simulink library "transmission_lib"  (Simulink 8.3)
settings: Solver=ode45  StartTime=0.0  StopTime=10.0  RelTol=1e-3
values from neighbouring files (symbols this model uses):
  dual_clutch = class_REVS_dual_clutch    [class_REVS_DCT_transmission.m]
  electric = class_REVS_electric(engine)    [electric_standard_car.m]
  gear = class_REVS_gearbox    [class_REVS_AMT_transmission.m]    (also in class_REVS_AT_transmission.m; class_REVS_CVT_transmission.m)
  torque_converter = class_REVS_torque_converter    [class_REVS_AT_transmission.m]    (also in class_REVS_CVT_transmission.m)
  transmission = class_REVS_AT_transmission    [transmission_6AT.m]    (also in transmission_8DCT.m = class_REVS_DCT_transmission; transmission_CVT.m = class_REVS_CVT_transmission)
undefined symbols (not defined in the file or in its folder): clutch, convert, gear_strategy, InitialSpeed_radps, LoadSource, SpeedSource, Value
libraries: general_lib x129, simulink x57, transmission_lib x50, audit_lib x11
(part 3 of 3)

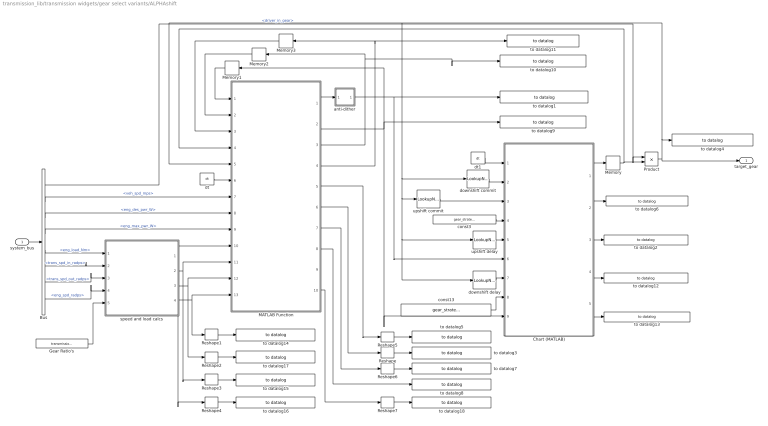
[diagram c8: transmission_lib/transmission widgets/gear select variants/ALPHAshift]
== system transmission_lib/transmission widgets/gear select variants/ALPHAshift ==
  system_bus : Inport
  Bus : BusSelector  OutputSignals=driver.driver_in_gear,vehicle.veh_spd_mps,powertrain.engine.eng_des_pwr_W,powertrain.engine.eng_max_pwr_W,powertrain.engine.eng_load_Nm,powertrain.trans.core.trans_spd_in_radps,powertrain.trans.core.trans_spd_out_radps,powertrain.engine.eng_spd_radps
  Chart (MATLAB) : Stateflow chart  TreatAsAtomicUnit=on
  Gear Ratio's : Constant  Value=transmission.gear.ratio  VectorParams1D=off
  MATLAB Function : MATLAB Function  TreatAsAtomicUnit=on
  Memory{,1..3} (4 alike) : Memory
  Product : Product
  Reshape{,1..7} (8 alike) : Reshape
  anti-dither : Subsystem
  const13 : Constant  Value=gear_strategy.disable_cost_saving_downshifts
  const3 : Constant  Value=gear_strategy.launch_gear_num
  downshift commit : LookupNDDirect  NumberOfTableDimensions=1  Table=gear_strategy.downshift_commit_secs
  downshift delay : LookupNDDirect  NumberOfTableDimensions=1  Table=gear_strategy.downshift_delay_secs
  dt : general_lib/dt
  dt1 : general_lib/dt
  speed and load calcs : Subsystem
  to datalog1 : general_lib/to datalog  VarName=ALPHAshift.desired_gear_num  WorkspaceName=datalog__ALPHAshift__desired_gear_num  VerboseLevel=1  VerboseSignal=REVS.verbose
  to datalog10 : general_lib/to datalog  VarName=ALPHAshift.kickdown_timer  WorkspaceName=datalog__ALPHAshift__kickdown_timer  VerboseLevel=2  VerboseSignal=REVS.verbose
  to datalog11 : general_lib/to datalog  VarName=ALPHAshift.kickdown_ratio  WorkspaceName=datalog__ALPHAshift__kickdown_ratio  VerboseLevel=2  VerboseSignal=REVS.verbose
  to datalog12 : general_lib/to datalog  VarName=ALPHAshift.shift_delay_timer  WorkspaceName=datalog__ALPHAshift__shift_delay_timer  VerboseLevel=2  VerboseSignal=REVS.verbose
  to datalog13 : general_lib/to datalog  VarName=ALPHAshift.in_gear_timer  WorkspaceName=datalog__ALPHAshift__in_gear_timer  VerboseLevel=2  VerboseSignal=REVS.verbose
  to datalog14 : general_lib/to datalog  VarName=ALPHAshift.gear_avail_torque_Nm  WorkspaceName=datalog__ALPHAshift__gear_avail_torque_Nm  VerboseLevel=2  VerboseSignal=REVS.verbose
  to datalog15 : general_lib/to datalog  VarName=ALPHAshift.gear_speed_radps  WorkspaceName=datalog__ALPHAshift__gear_speed_radps  VerboseLevel=2  VerboseSignal=REVS.verbose
  to datalog16 : general_lib/to datalog  VarName=ALPHAshift.gear_torque_Nm  WorkspaceName=datalog__ALPHAshift__gear_torque_Nm  VerboseLevel=2  VerboseSignal=REVS.verbose
  to datalog17 : general_lib/to datalog  VarName=ALPHAshift.gear_cost  WorkspaceName=datalog__ALPHAshift__gear_cost  VerboseLevel=2  VerboseSignal=REVS.verbose
  to datalog18 : general_lib/to datalog  VarName=ALPHAshift.kickdown_disability_code  WorkspaceName=datalog__ALPHAshift__kickdown_disability_code  VerboseLevel=2  VerboseSignal=REVS.verbose
  to datalog2 : general_lib/to datalog  VarName=ALPHAshift.shift_reason  WorkspaceName=datalog__ALPHAshift__shift_reason  VerboseLevel=1  VerboseSignal=REVS.verbose
  to datalog3 : general_lib/to datalog  VarName=ALPHAshift.disability_code  WorkspaceName=datalog__ALPHAshift__disability_code  VerboseLevel=2  VerboseSignal=REVS.verbose
  to datalog4 : general_lib/to datalog  VarName=ALPHAshift.current_gear_num  WorkspaceName=datalog__ALPHAshift__current_gear_num  VerboseLevel=1  VerboseSignal=REVS.verbose
  to datalog5 : general_lib/to datalog  VarName=ALPHAshift.gear_available  WorkspaceName=datalog__ALPHAshift__gear_available  VerboseLevel=2  VerboseSignal=REVS.verbose
  to datalog6 : general_lib/to datalog  VarName=ALPHAshift.shift_type  WorkspaceName=datalog__ALPHAshift__shift_type  VerboseLevel=1  VerboseSignal=REVS.verbose
  to datalog7 : general_lib/to datalog  VarName=ALPHAshift.better_fuel_gear  WorkspaceName=datalog__ALPHAshift__better_fuel_gear  VerboseLevel=1  VerboseSignal=REVS.verbose
  to datalog8 : general_lib/to datalog  VarName=ALPHAshift.min_fuel_gear  WorkspaceName=datalog__ALPHAshift__min_fuel_gear  VerboseLevel=1  VerboseSignal=REVS.verbose
  to datalog9 : general_lib/to datalog  VarName=ALPHAshift.desired_shift_reason  WorkspaceName=datalog__ALPHAshift__desired_shift_reason  VerboseLevel=1  VerboseSignal=REVS.verbose
  upshift commit : LookupNDDirect  NumberOfTableDimensions=1  Table=gear_strategy.upshift_commit_secs
  upshift delay : LookupNDDirect  NumberOfTableDimensions=1  Table=gear_strategy.upshift_delay_secs
  target_gear : Outport
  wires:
  Reshape6/1 -> to datalog7/1
  Reshape5/1 -> to datalog5/1
  MATLAB Function/1(desired_gear_num) -> anti-dither/1(raw)
  anti-dither/1(out) -> Chart (MATLAB)/6(desired_gear_num), to datalog1/1
  Reshape1/1 -> to datalog14/1
  Reshape3/1 -> to datalog15/1
  Reshape4/1 -> to datalog16/1
  Reshape/1 -> to datalog3/1
  speed and load calcs/4(gear_avail_trq_Nm) -> MATLAB Function/13(gear_avail_trq_Nm), Reshape1/1
  MATLAB Function/8(min_cost_gear) -> to datalog8/1
  MATLAB Function/7(better_cost_gear) -> Reshape6/1
  Chart (MATLAB)/1(command_gear_num) -> Memory/1
  Bus/2 -> MATLAB Function/7(vehicle_spd_mps)  "<veh_spd_mps>"
  dt/1 -> MATLAB Function/6(dt)
  speed and load calcs/3(gear_cost) -> Reshape2/1, MATLAB Function/12(gear_cost)
  system_bus/1 -> Bus/1
  Product/1 -> target_gear/1, to datalog4/1, downshift delay/1, upshift delay/1, upshift commit/1, downshift commit/1, MATLAB Function/5(current_gear_num)
  Chart (MATLAB)/3(shift_reason) -> to datalog2/1
  MATLAB Function/6(gear_disability_code) -> Reshape/1
  MATLAB Function/5(gear_available) -> Reshape5/1
  Chart (MATLAB)/2(previous_shift_type) -> to datalog6/1
  Bus/3 -> MATLAB Function/8(driver_des_pwr_W)  "<eng_des_pwr_W>"
  Bus/4 -> MATLAB Function/9(engine_max_pwr_W)  "<eng_max_pwr_W>"
  Memory/1 -> Product/2, MATLAB Function/4(command_gear_num)
  Bus/1 -> Product/1  "<driver_in_gear>"
  dt1/1 -> Chart (MATLAB)/1(dt)
  downshift delay/1 -> Chart (MATLAB)/7(downshift_delay_secs)
  upshift commit/1 -> Chart (MATLAB)/3(upshift_min_duration_secs)
  downshift commit/1 -> Chart (MATLAB)/2(downshift_min_duration_secs)
  upshift delay/1 -> Chart (MATLAB)/5(upshift_delay_secs)
  const13/1 -> Chart (MATLAB)/8(legacy_downshift_mode)
  const3/1 -> Chart (MATLAB)/4(launch_gear_num)
  MATLAB Function/2(desired_shift_reason) -> Chart (MATLAB)/9(desired_shift_reason), Memory1/1, to datalog9/1
  Memory1/1 -> MATLAB Function/1(desired_shift_reason_prev)
  MATLAB Function/3(kickdown_timer) -> to datalog10/1, Memory2/1
  Memory2/1 -> MATLAB Function/2(kickdown_timer_prev)
  Memory3/1 -> MATLAB Function/3(kickdown_ratio_prev)
  MATLAB Function/4(kickdown_ratio) -> Memory3/1, to datalog11/1
  speed and load calcs/2(gear_spd_radps) -> MATLAB Function/11(gear_spd_radps), Reshape3/1
  Bus/5 -> speed and load calcs/1(eng_load_Nm)  "<eng_load_Nm>"
  Bus/6 -> speed and load calcs/2(trans_spd_in_radps)  "<trans_spd_in_radps>"
  Bus/7 -> speed and load calcs/3(trans_spd_out_radps)  "<trans_spd_out_radps>"
  Bus/8 -> speed and load calcs/4(eng_spd_radps)  "<eng_spd_radps>"
  Gear Ratio's/1 -> speed and load calcs/5(trans_gear_ratios)
  speed and load calcs/1(gear_trq_Nm) -> MATLAB Function/10(gear_trq_Nm), Reshape4/1
  Chart (MATLAB)/4(shift_delay_timer) -> to datalog12/1
  Chart (MATLAB)/5(in_gear_timer) -> to datalog13/1
  Reshape2/1 -> to datalog17/1
  Reshape7/1 -> to datalog18/1
  MATLAB Function/10(kickdown_disability_code) -> Reshape7/1

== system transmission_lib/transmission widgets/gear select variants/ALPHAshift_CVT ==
  system_bus : Inport
  Bus Selector : BusSelector  OutputSignals=powertrain.trans.core.trans_spd_out_radps,driver.driver_in_gear,powertrain.engine.eng_des_pwr_W
  MinMax : MinMax  Function=max  Inputs=2
  Product2 : Product  Inputs=**
  Product4 : Product  Inputs=*/
  Saturation5 : Saturate  UpperLimit=max(transmission.gear.ratio)  LowerLimit=min(transmission.gear.ratio(2:end))
  Transfer Fcn : TransferFcn  Denominator=[0.0 1]
  eps : Saturate  UpperLimit=Inf  LowerLimit=eps
  min BSFC speed : Lookup_n-D  NumberOfTableDimensions=1  BreakpointsForDimension1=transmission.gear_strategy.min_bsfc_power_W  Table=transmission.gear_strategy.min_bsfc_speed_rapds  ExtrapMethod=Clip  InternalRulePriority=Speed  RndMeth=Simplest
  min speed table : general_lib/dynamic lookup  LookupStructure=transmission.gear_strategy.min_speed_radps  InterpMethod=Linear  ExtrapMethod=Clip  DiagnosticForOutOfRangeInput=Warning  IndexSearchMethod=Linear search  BeginIndexSearchUsingPreviousIndexResult=on  SupportTunableTableSize=off  LookupStructureEval=|
      | LookupStructure =
      | 
      |      []
  to datalog1 : general_lib/to datalog  VarName=cvtshift.target_ratio  WorkspaceName=datalog__cvtshift__target_ratio  VerboseLevel=3  VerboseSignal=REVS.verbose
  to datalog8 : general_lib/to datalog  VarName=cvtshift.target_speed_radps  WorkspaceName=datalog__cvtshift__target_speed_radps  VerboseLevel=3  VerboseSignal=REVS.verbose
  target_gear : Outport
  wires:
  system_bus/1 -> min speed table/1, Bus Selector/1
  Bus Selector/1 -> eps/1  "<trans_spd_out_radps>"
  Bus Selector/3 -> min BSFC speed/1  "<eng_des_pwr_W>"
  Product4/1 -> Saturation5/1
  Saturation5/1 -> Product2/2
  eps/1 -> Product4/2
  Bus Selector/2 -> Product2/1  "<driver_in_gear>"
  Product2/1 -> Transfer Fcn/1
  Transfer Fcn/1 -> to datalog1/1, target_gear/1
  min BSFC speed/1 -> MinMax/1
  min speed table/1 -> MinMax/2
  MinMax/1 -> to datalog8/1, Product4/1

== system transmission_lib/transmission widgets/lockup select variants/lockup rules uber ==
  gear_number : Inport
  system_bus : Inport  Port=2
  Bus Creator1 : BusCreator  Inputs=3
  Data Type Conversion : DataTypeConversion
  Detect Decrease : simulink/Logic and Bit Operations/Detect Decrease  vinit=0.0  InputProcessing=Inherited  OutDataTypeStr=boolean
  Detect Increase : simulink/Logic and Bit Operations/Detect Increase  vinit=0.0  InputProcessing=Inherited  OutDataTypeStr=boolean
  Logical Operator2 : Logic  Operator=NAND  AllPortsSameDT=off  OutDataTypeStr=boolean
  Logical Operator3 : Logic  Operator=NOT  AllPortsSameDT=off  OutDataTypeStr=boolean
  Logical Operator6 : Logic  Operator=NAND  AllPortsSameDT=off  OutDataTypeStr=boolean
  Logical Operator8 : Logic  Operator=OR  AllPortsSameDT=off  OutDataTypeStr=boolean
  Logical Operator9 : Logic  Inputs=5  AllPortsSameDT=off  OutDataTypeStr=boolean
  Memory : Memory
  Relational Operator : RelationalOperator  Operator=>  OutDataTypeStr=boolean  ZeroCross=off
  boolean integrator : general_lib/boolean integrator  UpperSaturationLimit=Inf  Normalize=off
  const1 : Constant  Value=transmission.tcc_strategy.lockup_allowed
  const3 : Constant  Value=transmission.tcc_strategy.lockup_delay_secs
  downshift unlock criteria : general_lib/dynamic equation  DynamicExpression=transmission.tcc_strategy.downshift_unlock_condition  DynamicExpressionEval=0
  lockup criteria : general_lib/dynamic equation  DynamicExpression=transmission.tcc_strategy.lock_condition  DynamicExpressionEval=(@gb_spd_out_radps > @table_lock_spd && @trans_curr_gear > transmission.tcc_strategy.always_unlock_gear ) || @trans_curr_gear >= transmission.tcc_strategy.always_lock_gear
  lockup table : general_lib/dynamic lookup  LookupStructure=transmission.tcc_strategy.lock_table  InterpMethod=Linear  ExtrapMethod=Clip  DiagnosticForOutOfRangeInput=Warning  IndexSearchMethod=Linear search  BeginIndexSearchUsingPreviousIndexResult=on  SupportTunableTableSize=off  LookupStructureEval=|
      | LookupStructure =
      | 
      |      []
  unlock criteria : general_lib/dynamic equation  DynamicExpression=transmission.tcc_strategy.unlock_condition  DynamicExpressionEval=(@gb_spd_out_radps < @table_unlock_spd && @trans_curr_gear < transmission.tcc_strategy.always_lock_gear ) || @trans_curr_gear <= transmission.tcc_strategy.always_unlock_gear
  unlock table : general_lib/dynamic lookup  LookupStructure=transmission.tcc_strategy.unlock_table  InterpMethod=Linear  ExtrapMethod=Clip  DiagnosticForOutOfRangeInput=Warning  IndexSearchMethod=Linear search  BeginIndexSearchUsingPreviousIndexResult=on  SupportTunableTableSize=off  LookupStructureEval=|
      | LookupStructure =
      | 
      |      []
  upshift unlock criteria : general_lib/dynamic equation  DynamicExpression=transmission.tcc_strategy.upshift_unlock_condition  DynamicExpressionEval=0
  lockup_cmd : Outport
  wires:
  Logical Operator6/1 -> Logical Operator9/2
  Logical Operator2/1 -> Logical Operator9/3
  Detect Increase/1 -> Logical Operator2/2
  system_bus/1 -> Bus Creator1/3, unlock table/1, lockup table/1, upshift unlock criteria/1, downshift unlock criteria/1  "system_bus"
  Logical Operator9/1 -> boolean integrator/1
  Logical Operator8/1 -> Logical Operator9/4
  const3/1 -> Relational Operator/2
  Detect Decrease/1 -> Logical Operator6/2
  gear_number/1 -> Detect Increase/1, Detect Decrease/1
  boolean integrator/1 -> Relational Operator/1
  const1/1 -> Logical Operator9/1
  Relational Operator/1 -> Data Type Conversion/1
  Data Type Conversion/1 -> lockup_cmd/1, Memory/1  "tcc_lockup_cmd_bool"
  unlock criteria/1 -> Logical Operator3/1
  downshift unlock criteria/1 -> Logical Operator6/1
  upshift unlock criteria/1 -> Logical Operator2/1
  Logical Operator3/1 -> Logical Operator9/5
  lockup table/1 -> Bus Creator1/1  "table_lock_spd"
  Bus Creator1/1 -> lockup criteria/1, unlock criteria/1
  unlock table/1 -> Bus Creator1/2  "table_unlock_spd"
  lockup criteria/1 -> Logical Operator8/2
  Memory/1 -> Logical Operator8/1

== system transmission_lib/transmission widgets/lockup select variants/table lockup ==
  gear_number : Inport
  system_bus : Inport  Port=2
  const : Constant  Value=transmission.tcc_strategy.lockup_allowed
  const2 : Constant  Value=transmission.tcc_strategy.lockup_delay_secs
  dt : general_lib/dt
  "lock map " : Lookup_n-D  BreakpointsForDimension1=transmission.tcc_strategy.lock_map_load  BreakpointsForDimension2=transmission.gear.number(2:end)  Table=transmission.tcc_strategy.lock_map_speed  RndMeth=Simplest
  lockup load select : transmission_lib/transmission widgets/load select  LoadSource=transmission.tcc_strategy.lockup_load_source
  lockup speed select : transmission_lib/transmission widgets/speed select  SpeedSource=transmission.tcc_strategy.lockup_speed_source
  tcc lockup : Stateflow chart  TreatAsAtomicUnit=on
  "unlock map " : Lookup_n-D  BreakpointsForDimension1=transmission.tcc_strategy.unlock_map_load  BreakpointsForDimension2=transmission.gear.number(2:end)  Table=transmission.tcc_strategy.unlock_map_speed  RndMeth=Simplest
  lockup_cmd : Outport
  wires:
  dt/1 -> tcc lockup/2(step_time)
  lockup speed select/1 -> tcc lockup/1(lock_spd)
  "unlock map "/1 -> tcc lockup/4(release_spd)
  "lock map "/1 -> tcc lockup/3(lockup_spd)
  tcc lockup/1(tcc_lockup) -> lockup_cmd/1  "tcc_lockup_cmd_bool"
  const/1 -> tcc lockup/5(lockup_allowed)
  lockup load select/1 -> "unlock map "/1, "lock map "/1
  const2/1 -> tcc lockup/6(lockup_delay_secs)
  system_bus/1 -> lockup load select/1, lockup speed select/1
  gear_number/1 -> "lock map "/2, "unlock map "/2

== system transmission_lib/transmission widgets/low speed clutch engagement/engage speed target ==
  curr : Inport
  Constant : Constant  Value=clutch.engage_speed_radps(1)
  Constant1 : Constant  Value=clutch.engage_speed_radps(end)
  Divide : Product  Inputs=*/
  Interp 0-1 : general_lib/Interp 0-1
  tgt : Outport
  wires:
  Constant/1 -> Interp 0-1/2
  Constant1/1 -> Interp 0-1/3, Divide/2
  Divide/1 -> Interp 0-1/1
  curr/1 -> Divide/1
  Interp 0-1/1 -> tgt/1

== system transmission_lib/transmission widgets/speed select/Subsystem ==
  veh_spd_mps : Inport
  Axle Speed (rad/sec) : Product  Inputs=/*
  Non Zero : Saturate  UpperLimit=Inf  LowerLimit=eps  ZeroCross=off
  Tire Radius (m) : Constant  Value=vehicle.drive_axle1.tire.radius_m
  wheel_spd_radps : Outport
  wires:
  Tire Radius (m)/1 -> Non Zero/1
  Axle Speed (rad/sec)/1 -> wheel_spd_radps/1
  Non Zero/1 -> Axle Speed (rad/sec)/1
  veh_spd_mps/1 -> Axle Speed (rad/sec)/2

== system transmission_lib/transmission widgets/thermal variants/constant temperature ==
  system_bus : Inport
  Bus Creator : BusCreator  Inputs=1
  Constant : Constant  Value=transmission.thermal.temperature_degC
  thermal_bus : Outport
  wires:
  Constant/1 -> Bus Creator/1  "trans_temp_degC"
  Bus Creator/1 -> thermal_bus/1

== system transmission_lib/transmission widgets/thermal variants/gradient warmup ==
  system_bus : Inport
  Bus Creator : BusCreator  Inputs=1
  Constant : Constant  Value=transmission.thermal.final_temperature_degC
  State-Space : StateSpace  A=-1/transmission.thermal.gradient_time_constant_sec  C=1/transmission.thermal.gradient_time_constant_sec  D=0  X0=transmission.thermal.initial_temperature_degC  ContinuousStateAttributes='temperature'
  thermal_bus : Outport
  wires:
  State-Space/1 -> Bus Creator/1  "trans_temp_degC"
  Bus Creator/1 -> thermal_bus/1
  Constant/1 -> State-Space/1

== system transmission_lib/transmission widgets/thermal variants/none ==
  system_bus : Inport
  thermal_bus : Outport

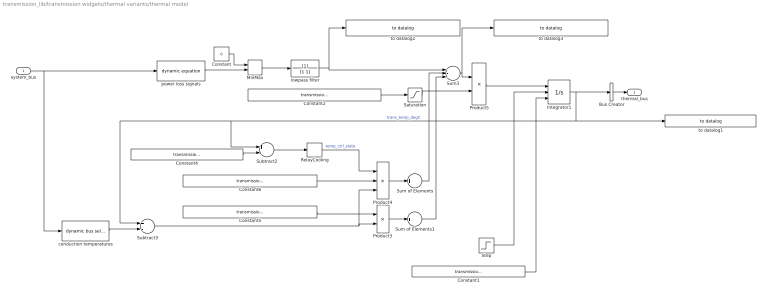
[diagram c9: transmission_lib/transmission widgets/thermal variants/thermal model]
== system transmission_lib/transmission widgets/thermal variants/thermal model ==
  system_bus : Inport
  Bus Creator : BusCreator  Inputs=1
  Constant : Constant  Value=0
  Constant1 : Constant  Value=transmission.thermal.initial_temperature_degC
  Constant2 : Constant  Value=transmission.thermal.capacity_JpK
  Constant4 : Constant  Value=transmission.thermal.target_temperature_degC
  Constant5 : Constant  Value=transmission.thermal.passive_conductance_WpK
  Constant6 : Constant  Value=transmission.thermal.cooling_conductance_WpK
  Integrator1 : Integrator  ExternalReset=level  InitialConditionSource=external  InitialCondition=transmission.thermal.initial_temperature_degC  ZeroCross=off
  MinMax : MinMax  Function=max  Inputs=2
  Product3 : Product  Inputs=**
  Product4 : Product  Inputs=***
  Product5 : Product  Inputs=*/
  RelayCooling : Relay  OnSwitchValue=1  OffSwitchValue=-1  ZeroCross=off
  Saturation : Saturate  UpperLimit=Inf  LowerLimit=eps
  Step : Step  Before=1  After=0  SampleTime=0  ZeroCross=off
  Subtract2 : Sum  Inputs=+-
  Subtract3 : Sum  Inputs=+-
  Sum of Elements : Sum  Inputs=+
  Sum of Elements1 : Sum  Inputs=+
  Sum3 : Sum  Inputs=+--
  conduction temperatures : general_lib/dynamic bus select  SignalList=transmission.thermal.conduction_temperatures
  lowpass filter : TransferFcn  Denominator=[1 1]
  power loss signals : general_lib/dynamic equation  DynamicExpression=transmission.thermal.power_loss_expr
  to datalog1 : general_lib/to datalog  VarName=transmission.temperature_C  WorkspaceName=datalog__transmission__temperature_C  VerboseLevel=2  VerboseSignal=REVS.verbose
  to datalog2 : general_lib/to datalog  VarName=transmission.thermal_loss_power_input_W  WorkspaceName=datalog__transmission__thermal_loss_power_input_W  VerboseLevel=2  VerboseSignal=REVS.verbose
  to datalog3 : general_lib/to datalog  VarName=transmission.thermal_net_power_W  WorkspaceName=datalog__transmission__thermal_net_power_W  VerboseLevel=2  VerboseSignal=REVS.verbose
  thermal_bus : Outport
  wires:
  Product4/1 -> Sum of Elements/1
  Product3/1 -> Sum of Elements1/1
  Sum of Elements/1 -> Sum3/2
  Sum of Elements1/1 -> Sum3/3
  Constant6/1 -> Product4/2
  Constant5/1 -> Product3/1
  Subtract3/1 -> Product3/2, Product4/3
  conduction temperatures/1 -> Subtract3/2
  Constant/1 -> MinMax/1
  power loss signals/1 -> MinMax/2
  system_bus/1 -> conduction temperatures/1, power loss signals/1
  lowpass filter/1 -> Sum3/1, to datalog2/1
  Product5/1 -> Integrator1/1
  Sum3/1 -> Product5/1, to datalog3/1
  Integrator1/1 -> Bus Creator/1, Subtract2/1, Subtract3/1, to datalog1/1  "trans_temp_degC"
  Constant2/1 -> Saturation/1
  Saturation/1 -> Product5/2
  MinMax/1 -> lowpass filter/1
  Bus Creator/1 -> thermal_bus/1
  Constant4/1 -> Subtract2/2
  RelayCooling/1 -> Product4/1  "temp_ctrl_state"
  Subtract2/1 -> RelayCooling/1
  Constant1/1 -> Integrator1/3
  Step/1 -> Integrator1/2

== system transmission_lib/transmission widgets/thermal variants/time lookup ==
  system_bus : Inport
  1-D Lookup Table : Lookup_n-D  NumberOfTableDimensions=1  BreakpointsForDimension1=transmission.thermal.temperature_time_sec  IndexSearchMethod=Linear search  BeginIndexSearchUsingPreviousIndexResult=on  Table=transmission.thermal.temperature_degC  ExtrapMethod=Clip  InternalRulePriority=Speed  RndMeth=Simplest
  Bus Creator : BusCreator  Inputs=1
  Bus Selector : BusSelector  OutputSignals=driver.cycle_pos_secs
  thermal_bus : Outport
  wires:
  Bus Selector/1 -> 1-D Lookup Table/1  "<cycle_pos_secs>"
  1-D Lookup Table/1 -> Bus Creator/1  "trans_temp_degC"
  Bus Creator/1 -> thermal_bus/1
  system_bus/1 -> Bus Selector/1

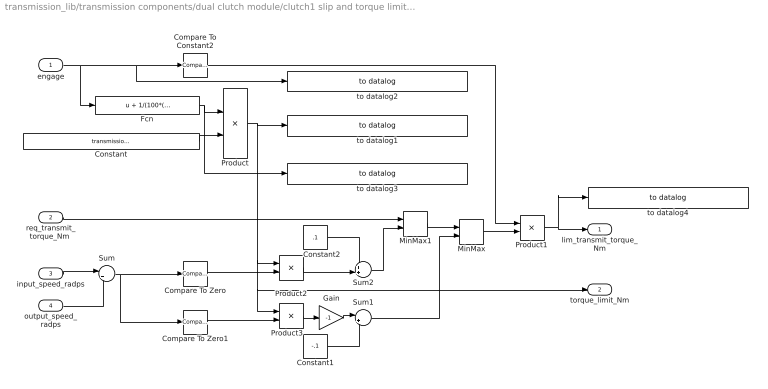
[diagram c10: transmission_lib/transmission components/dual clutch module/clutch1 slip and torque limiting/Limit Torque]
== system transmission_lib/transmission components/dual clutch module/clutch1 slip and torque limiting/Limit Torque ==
  engage : Inport
  "req_transmit_torque_Nm " : Inport  Port=2
  input_speed_radps : Inport  Port=3
  output_speed_radps : Inport  Port=4
  Compare To Constant2 : simulink/Logic and Bit Operations/Compare To Constant  relop=>  const=0  OutDataTypeStr=boolean
  Compare To Zero : simulink/Logic and Bit Operations/Compare To Zero  relop=>=  OutDataTypeStr=boolean  ZeroCross=off
  Compare To Zero1 : simulink/Logic and Bit Operations/Compare To Zero  relop=<=  OutDataTypeStr=boolean  ZeroCross=off
  Constant : Constant  Value=transmission.dual_clutch.torque_capacity_Nm
  Constant1 : Constant  Value=-.1
  Constant2 : Constant  Value=.1
  Fcn : Fcn  Expr=u + 1/(100*(1+eps-u))
  Gain : Gain  Gain=-1
  MinMax : MinMax  Function=max  Inputs=2  ZeroCross=off
  MinMax1 : MinMax  Inputs=2  ZeroCross=off
  Product{,1..3} (4 alike) : Product
  Sum : Sum  Inputs=|+-
  Sum1 : Sum  Inputs=|++
  Sum2 : Sum  Inputs=++|
  to datalog1 : general_lib/to datalog  VarName=transmission__clutch1_torque_limit_Nm  WorkspaceName=datalog__transmission__clutch1_torque_limit_Nm  VerboseLevel=3  VerboseSignal=REVS.verbose
  to datalog2 : general_lib/to datalog  VarName=transmission__clutch1_engage  WorkspaceName=datalog__transmission__clutch1_engage  VerboseLevel=1  VerboseSignal=REVS.verbose
  to datalog3 : general_lib/to datalog  VarName=transmission__clutch1_capacity_norm  WorkspaceName=datalog__transmission__clutch1_capacity_norm  VerboseLevel=3  VerboseSignal=REVS.verbose
  to datalog4 : general_lib/to datalog  VarName=transmission__clutch1_torque_Nm  WorkspaceName=datalog__transmission__clutch1_torque_Nm  VerboseLevel=3  VerboseSignal=REVS.verbose
  lim_transmit_torque_Nm : Outport
  torque_limit_Nm : Outport  Port=2
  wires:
  Fcn/1 -> Product/1, to datalog3/1
  Sum2/1 -> MinMax1/2
  Product3/1 -> Gain/1
  Constant2/1 -> Sum2/1
  Product2/1 -> Sum2/2
  Compare To Zero1/1 -> Product3/2
  Compare To Zero/1 -> Product2/2
  Sum/1 -> Compare To Zero/1, Compare To Zero1/1
  Sum1/1 -> MinMax/2
  Constant1/1 -> Sum1/2
  output_speed_radps/1 -> Sum/2
  input_speed_radps/1 -> Sum/1
  "req_transmit_torque_Nm "/1 -> MinMax1/1
  Gain/1 -> Sum1/1
  MinMax1/1 -> MinMax/1
  Constant/1 -> Product/2
  engage/1 -> Fcn/1, Compare To Constant2/1, to datalog2/1
  Product/1 -> to datalog1/1, torque_limit_Nm/1, Product3/1, Product2/1
  MinMax/1 -> Product1/2
  Product1/1 -> lim_transmit_torque_Nm/1, to datalog4/1
  Compare To Constant2/1 -> Product1/1

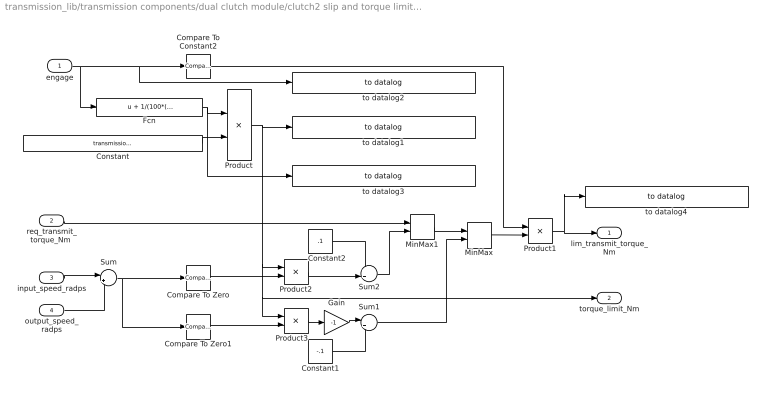
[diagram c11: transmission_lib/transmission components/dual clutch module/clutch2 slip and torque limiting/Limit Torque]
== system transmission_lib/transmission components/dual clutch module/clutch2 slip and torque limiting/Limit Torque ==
  engage : Inport
  "req_transmit_torque_Nm " : Inport  Port=2
  input_speed_radps : Inport  Port=3
  output_speed_radps : Inport  Port=4
  Compare To Constant2 : simulink/Logic and Bit Operations/Compare To Constant  relop=>  const=0  OutDataTypeStr=boolean
  Compare To Zero : simulink/Logic and Bit Operations/Compare To Zero  relop=>=  OutDataTypeStr=boolean  ZeroCross=off
  Compare To Zero1 : simulink/Logic and Bit Operations/Compare To Zero  relop=<=  OutDataTypeStr=boolean  ZeroCross=off
  Constant : Constant  Value=transmission.dual_clutch.torque_capacity_Nm
  Constant1 : Constant  Value=-.1
  Constant2 : Constant  Value=.1
  Fcn : Fcn  Expr=u + 1/(100*(1+eps-u))
  Gain : Gain  Gain=-1
  MinMax : MinMax  Function=max  Inputs=2  ZeroCross=off
  MinMax1 : MinMax  Inputs=2  ZeroCross=off
  Product{,1..3} (4 alike) : Product
  Sum : Sum  Inputs=|+-
  Sum1 : Sum  Inputs=|++
  Sum2 : Sum  Inputs=++|
  to datalog1 : general_lib/to datalog  VarName=transmission__clutch2_torque_limit_Nm  WorkspaceName=datalog__transmission__clutch2_torque_limit_Nm  VerboseLevel=3  VerboseSignal=REVS.verbose
  to datalog2 : general_lib/to datalog  VarName=transmission__clutch2_engage  WorkspaceName=datalog__transmission__clutch2_engage  VerboseLevel=1  VerboseSignal=REVS.verbose
  to datalog3 : general_lib/to datalog  VarName=transmission__clutch2_capacity_norm  WorkspaceName=datalog__transmission__clutch2_capacity_norm  VerboseLevel=3  VerboseSignal=REVS.verbose
  to datalog4 : general_lib/to datalog  VarName=transmission__clutch2_torque_Nm  WorkspaceName=datalog__transmission__clutch2_torque_Nm  VerboseLevel=3  VerboseSignal=REVS.verbose
  lim_transmit_torque_Nm : Outport
  torque_limit_Nm : Outport  Port=2
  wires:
  Fcn/1 -> Product/1, to datalog3/1
  Sum2/1 -> MinMax1/2
  Product3/1 -> Gain/1
  Constant2/1 -> Sum2/1
  Product2/1 -> Sum2/2
  Compare To Zero1/1 -> Product3/2
  Compare To Zero/1 -> Product2/2
  Sum/1 -> Compare To Zero/1, Compare To Zero1/1
  Sum1/1 -> MinMax/2
  Constant1/1 -> Sum1/2
  output_speed_radps/1 -> Sum/2
  input_speed_radps/1 -> Sum/1
  "req_transmit_torque_Nm "/1 -> MinMax1/1
  Gain/1 -> Sum1/1
  MinMax1/1 -> MinMax/1
  Constant/1 -> Product/2
  engage/1 -> Compare To Constant2/1, to datalog2/1, Fcn/1
  Product/1 -> to datalog1/1, torque_limit_Nm/1, Product3/1, Product2/1
  MinMax/1 -> Product1/2
  Product1/1 -> lim_transmit_torque_Nm/1, to datalog4/1
  Compare To Constant2/1 -> Product1/1

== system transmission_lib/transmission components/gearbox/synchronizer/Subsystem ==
  engage : Inport
  spd_out : Inport  Port=2
  spd_in : Inport  Port=3
  Compare To Constant1 : simulink/Logic and Bit Operations/Compare To Constant  relop=<=  const=1e-3  OutDataTypeStr=boolean  ZeroCross=off
  Compare To Constant2 : simulink/Logic and Bit Operations/Compare To Constant  relop=<=  const=1e-3  OutDataTypeStr=boolean  ZeroCross=off
  Compare To Constant3 : simulink/Logic and Bit Operations/Compare To Constant  relop=>  const=0  OutDataTypeStr=boolean  ZeroCross=off
  Compare To Constant4 : simulink/Logic and Bit Operations/Compare To Constant  relop===  const=1  OutDataTypeStr=boolean
  Logical Operator : Logic  Operator=OR  AllPortsSameDT=off  OutDataTypeStr=boolean
  Logical Operator1 : Logic  Inputs=3  AllPortsSameDT=off  OutDataTypeStr=boolean
  Memory2 : Memory
  lockup : Outport
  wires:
  Compare To Constant4/1 -> Logical Operator/1
  Memory2/1 -> Logical Operator/2
  Compare To Constant1/1 -> Logical Operator1/2
  Compare To Constant2/1 -> Logical Operator1/3
  engage/1 -> Compare To Constant3/1, Compare To Constant4/1
  Logical Operator/1 -> lockup/1
  spd_out/1 -> Compare To Constant1/1
  spd_in/1 -> Compare To Constant2/1
  Logical Operator1/1 -> Memory2/1
  Compare To Constant3/1 -> Logical Operator1/1

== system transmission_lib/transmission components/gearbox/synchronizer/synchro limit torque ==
  engage : Inport
  "req_transmit_torque_Nm " : Inport  Port=2
  input_speed_radps : Inport  Port=3
  output_speed_radps : Inport  Port=4
  Compare To Constant2 : simulink/Logic and Bit Operations/Compare To Constant  relop=>  const=0  OutDataTypeStr=boolean
  Compare To Zero : simulink/Logic and Bit Operations/Compare To Zero  relop=>=  OutDataTypeStr=boolean
  Compare To Zero1 : simulink/Logic and Bit Operations/Compare To Zero  relop=<=  OutDataTypeStr=boolean
  Constant : Constant  Value=.1
  Constant1 : Constant  Value=-.1
  Constant2 : Constant  Value=inf
  Constant3 : Constant  Value=-inf
  MinMax : MinMax  Function=max  Inputs=2  ZeroCross=off
  MinMax1 : MinMax  Inputs=2  ZeroCross=off
  Product : Product
  Product1 : Product
  Product2 : Product
  Sum : Sum  Inputs=|+-
  Sum1 : Sum  Inputs=|++
  Sum2 : Sum  Inputs=++|
  lim_transmit_torque_Nm : Outport
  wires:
  Sum2/1 -> MinMax1/2
  Sum/1 -> Compare To Zero/1, Compare To Zero1/1
  Compare To Constant2/1 -> Product1/1
  output_speed_radps/1 -> Sum/2
  input_speed_radps/1 -> Sum/1
  MinMax1/1 -> MinMax/1
  engage/1 -> Compare To Constant2/1
  MinMax/1 -> Product1/2
  "req_transmit_torque_Nm "/1 -> MinMax1/1
  Product1/1 -> lim_transmit_torque_Nm/1
  Sum1/1 -> MinMax/2
  Constant1/1 -> Sum1/2
  Constant/1 -> Sum2/1
  Compare To Zero/1 -> Product/2
  Compare To Zero1/1 -> Product2/1
  Constant3/1 -> Product2/2
  Constant2/1 -> Product/1
  Product2/1 -> Sum1/1
  Product/1 -> Sum2/2

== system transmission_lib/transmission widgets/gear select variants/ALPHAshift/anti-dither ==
  raw : Inport
  Abs : Abs
  Memory : Memory
  Rounding Function : Rounding  Operator=round
  Sum : Sum  Inputs=|+-
  Switch : Switch  Criteria=u2 > Threshold  Threshold=.66
  low pass filter : TransferFcn  Denominator=[0.02 1]
  to datalog17 : general_lib/to datalog  VarName=ALPHAshift.filtered_desired_gear_num  WorkspaceName=datalog__ALPHAshift__filtered_desired_gear_num  VerboseLevel=3  VerboseSignal=REVS.verbose
  to datalog18 : general_lib/to datalog  VarName=ALPHAshift.raw_desired_gear_num  WorkspaceName=datalog__ALPHAshift__raw_desired_gear_num  VerboseLevel=3  VerboseSignal=REVS.verbose
  out : Outport
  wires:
  Abs/1 -> Switch/2
  Memory/1 -> Switch/3, Sum/2
  Sum/1 -> Abs/1
  Switch/1 -> Memory/1, out/1
  Rounding Function/1 -> Switch/1
  low pass filter/1 -> to datalog17/1, Sum/1, Rounding Function/1
  raw/1 -> low pass filter/1, to datalog18/1

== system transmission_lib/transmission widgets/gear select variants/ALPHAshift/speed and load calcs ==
  eng_load_Nm : Inport
  trans_spd_in_radps : Inport  Port=2
  trans_spd_out_radps : Inport  Port=3
  eng_spd_radps : Inport  Port=4
  trans_gear_ratios : Inport  Port=5
  Logical Operator : Logic  Operator=NOT  AllPortsSameDT=off  OutDataTypeStr=boolean
  MinMax : MinMax  Inputs=2  ZeroCross=off
  MinMax1 : MinMax  Function=max  ZeroCross=off
  MinMax2 : MinMax  Function=max  Inputs=2  ZeroCross=off
  Product1 : Product  Inputs=***/
  Product2 : Product  Inputs=***
  Product3 : Product  Inputs=*/
  Product4 : Product  Inputs=***/
  Product5 : Product  Inputs=**
  Sum : Sum  Inputs=|++
  cost map : Lookup_n-D  BreakpointsForDimension1=gear_strategy.cost_map_torque_Nm  BreakpointsForDimension2=gear_strategy.cost_map_speed_radps  IndexSearchMethod=Linear search  BeginIndexSearchUsingPreviousIndexResult=on  Table=gear_strategy.cost_map  ExtrapMethod=Clip  UseLastTableValue=on  RndMeth=Simplest
  eps1 : Saturate  UpperLimit=Inf  LowerLimit=eps
  eps2 : Saturate  UpperLimit=Inf  LowerLimit=eps  ZeroCross=off
  eps3 : Saturate  UpperLimit=Inf  LowerLimit=eps
  max input torque : Lookup_n-D  NumberOfTableDimensions=1  BreakpointsForDimension1=gear_strategy.max_input_torque_speeds_radps  IndexSearchMethod=Linear search  BeginIndexSearchUsingPreviousIndexResult=on  Table=gear_strategy.max_input_torque_curve_Nm  ExtrapMethod=Clip  UseLastTableValue=on  RndMeth=Simplest
  non-neutral gears vector : simulink/Logic and Bit Operations/Compare To Zero  relop=~=  OutDataTypeStr=boolean
  non-neutral gears vector1 : simulink/Logic and Bit Operations/Compare To Zero  relop=~=  OutDataTypeStr=boolean
  speed mask : Constant  Value=gear_strategy.use_engine_speed_mask
  gear_trq_Nm : Outport
  gear_spd_radps : Outport  Port=2
  gear_cost : Outport  Port=3
  gear_avail_trq_Nm : Outport  Port=4
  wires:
  MinMax2/1 -> Product4/2
  speed mask/1 -> Product4/1, Logical Operator/1
  Logical Operator/1 -> Product2/3
  cost map/1 -> gear_cost/1
  non-neutral gears vector1/1 -> Product5/2
  Product5/1 -> gear_avail_trq_Nm/1
  max input torque/1 -> Product5/1
  trans_spd_out_radps/1 -> Product2/1, eps2/1
  trans_spd_in_radps/1 -> Product3/1, MinMax2/1
  MinMax1/1 -> MinMax/1
  MinMax/1 -> eps3/1
  Product3/1 -> MinMax/2
  eps2/1 -> Product3/2
  Product1/1 -> gear_trq_Nm/1, cost map/1  "engine_loads"
  Sum/1 -> gear_spd_radps/1, eps1/1, cost map/2, max input torque/1  "speeds"
  trans_gear_ratios/1 -> non-neutral gears vector1/1, Product4/3, Product2/2, non-neutral gears vector/1, MinMax1/1
  non-neutral gears vector/1 -> Product1/2
  eps1/1 -> Product1/4
  eng_load_Nm/1 -> Product1/1
  eng_spd_radps/1 -> MinMax2/2, Product1/3
  eps3/1 -> Product4/4
  Product2/1 -> Sum/1  "speeds"
  Product4/1 -> Sum/2  "engine_speeds"

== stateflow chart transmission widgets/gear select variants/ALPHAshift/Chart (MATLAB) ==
  state gear_command_timer
    entry:
    command_gear_num = launch_gear_num;
    shift_delay_timer = 0;
    in_gear_timer = 0;
    previous_shift_type = -1;
    during:
    % update timers
    shift_delay_timer = shift_delay_timer + dt;
    in_gear_timer = in_gear_timer + dt;
    state downshift_delay
    state upshift_delay
    state in_gear
      exit:
      shift_delay_timer = 0;
    (default) -> in_gear
    in_gear -> upshift_delay : [desired_gear_num > command_gear_num]
    in_gear -> downshift_delay : [desired_gear_num < command_gear_num]
    upshift_delay -> in_gear : [desired_gear_num <= command_gear_num]
    downshift_delay -> in_gear : [desired_gear_num >= command_gear_num]
    upshift_delay -> in_gear : [(shift_delay_timer >= upshift_delay_secs && ... (in_gear_timer > downshift_min_duration_secs && previous_shift_type == -1 || ... in_gear_timer > upshift_min_duration_secs && previous_shift_type == +1) ) || ... (shift_delay_timer >= upshift_delay_secs/10 && desired_shift_reason == 4)]   {command_gear_num = desired_gear_num; in_gear_timer = 0; previous_shift_type = +1; shift_reason = desired_shift_reason}
    downshift_delay -> in_gear : [shift_delay_timer >= downshift_delay_secs && ... (in_gear_timer > downshift_min_duration_secs && previous_shift_type == -1 || ... in_gear_timer > upshift_min_duration_secs && previous_shift_type == +1) || ... legacy_downshift_mode && (desired_shift_reason ~= 3) ]    {command_gear_num = desired_gear_num; in_gear_timer = 0; previous_shift_type = -1; shift_reason = desired_shift_reason}
  (default) -> gear_command_timer

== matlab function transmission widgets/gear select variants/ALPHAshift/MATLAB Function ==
 function [  desired_gear_num, ...
            desired_shift_reason, ...
            kickdown_timer, ...
            kickdown_ratio, ...
            gear_available, ...
            gear_disability_code, ...
            better_cost_gear, ...
            min_cost_gear, ... 
   kickdown_gear_available, ...
            kickdown_disability_code ...
          ] = ...
fcn(gear_strategy, ...
    desired_shift_reason_prev, ...
    kickdown_timer_prev, ...
    kickdown_ratio_prev, ...
    command_gear_num, ...
    current_gear_num, ...
    dt, ...
    vehicle_spd_mps, ...
    driver_des_pwr_W, ...
    engine_max_pwr_W, ...
    gear_trq_Nm, ...
    gear_spd_radps, ...
    gear_cost, ...
    gear_avail_trq_Nm) ...

% entry:
desired_shift_reason    = desired_shift_reason_prev;
kickdown_timer          = kickdown_timer_prev;
current_gear_index      = current_gear_num+1;
desired_gear_num        = current_gear_num; % init desired gear to current gear

num_gear_indices = length( gear_avail_trq_Nm );
gear_indices = reshape((1:num_gear_indices), size(gear_avail_trq_Nm));
gear_nums = gear_indices-1;

gear_avail_trq_Nm = gear_avail_trq_Nm .* (gear_nums > 0); % no torque available in neutral

% define which gears meet speed and torque boundary conditions:
gear_disability_code =  (gear_spd_radps < gear_strategy.min_speed_radps) * 1 + ...
                        (gear_spd_radps > gear_strategy.max_speed_radps) * 2 + ...
                        (gear_avail_trq_Nm < gear_trq_Nm) * 4 + ...
                        ((gear_nums > current_gear_num) & (gear_spd_radps < gear_strategy.upshift_min_speed_radps)) * 8 + ...
                        ((gear_nums > current_gear_num) & (gear_avail_trq_Nm < (gear_trq_Nm * gear_strategy.upshift_min_torque_reserve_ratio(current_gear_index)))) * 16 + ...
                        ((gear_nums < current_gear_num) & (gear_spd_radps > gear_strategy.downshift_max_speed_radps)) * 32 + ...;
                        (gear_strategy.restrict_skip_shifts & (abs(current_gear_num - gear_nums) > 1)) * 64 + ...
                        (gear_strategy.restrict_shift_parity & (mod(gear_nums,2) == mod(current_gear_num,2)) & (gear_nums ~= current_gear_num)) * 128 + ...
                        (gear_avail_trq_Nm == 0) * 256;

gear_available = (gear_disability_code == 0);

if isempty(gear_cost(gear_available & (gear_nums > 0)))
    min_fuel_gear_index = 2;
    min_cost_gear = 1;
else
    [~, min_index] = min(gear_cost(gear_available & (gear_nums > 0)));
    gear_indices_available = gear_indices(gear_available  & (gear_nums > 0));
    min_fuel_gear_index = gear_indices_available(min_index);
    min_cost_gear = gear_nums(min_fuel_gear_index);
end

% create binary vector of all gear indices that have better fuel
% cost and meet boundary conditions...
better_cost_gear = gear_available & (gear_cost < (gear_cost(current_gear_index) / gear_strategy.required_cost_benefit_ratio(current_gear_index)));

% calculate non-fuel-based shift points:
kickdown_ratio = max(0,driver_des_pwr_W/max(1,engine_max_pwr_W));
%future_kickdown_ratio = kickdown_ratio + (kickdown_ratio - kickdown_ratio_prev) * 1/dt;

if better_cost_gear(min_fuel_gear_index) && ...
        (min_fuel_gear_index ~= current_gear_index) && ...
        ( kickdown_ratio < gear_strategy.kickdown_trigger_ratio(current_gear_index) )
    if (min_fuel_gear_index > current_gear_index)
        desired_gear_num = min_cost_gear;
        desired_shift_reason = 1 + gear_disability_code(current_gear_index)/10;
    elseif (min_fuel_gear_index < current_gear_index) && (gear_strategy.disable_cost_saving_downshifts == false)
        desired_gear_num = min_cost_gear;
        desired_shift_reason = 2 + gear_disability_code(current_gear_index)/10;
    end
end


kickdown_disability_code = ...
    (gear_spd_radps >= gear_strategy.downshift_max_speed_radps) * 32 + ...	% Shared with codes above
	(gear_strategy.restrict_skip_shifts & (abs(current_gear_num - gear_nums) > 1)) * 64 + ...	% Shared with codes above
    (gear_strategy.restrict_shift_parity & (mod(gear_nums,2) == mod(current_gear_num,2))) * 128 + ...;	% Shared with codes above
	(gear_nums < (current_gear_num - gear_strategy.kickdown_max_increment)) * 256 + ...
    (gear_nums < gear_strategy.kickdown_min_gear) * 512 +...
	(gear_nums >= current_gear_num) * 1024;
kickdown_gear_available = (kickdown_disability_code == 0);

if  ( kickdown_ratio >= gear_strategy.kickdown_trigger_ratio(current_gear_index) ) && any(kickdown_gear_available)
    kickdown_timer = kickdown_timer + dt;
else
    kickdown_timer = 0;
end

if any(kickdown_gear_available & gear_available) && kickdown_timer >= gear_strategy.kickdown_delay_secs(current_gear_index)
    
    kickdown_power_available = ((gear_spd_radps .* gear_avail_trq_Nm - driver_des_pwr_W) > 0) & kickdown_gear_available ;
	
	if any(kickdown_power_available )
		desired_gear_num = max( gear_nums( kickdown_power_available ) );
	else
		desired_gear_num = min( gear_nums( kickdown_gear_available ) );
	end
	
    desired_shift_reason = 3;
end

if (gear_spd_radps(current_gear_index) > gear_strategy.max_speed_radps(current_gear_index)) 
	max_speed_upshift_gear_index = min(num_gear_indices, current_gear_index + gear_strategy.max_speed_shift_increment(current_gear_index));
	
	if  (gear_disability_code(max_speed_upshift_gear_index) < 256)
		desired_gear_num = command_gear_num + gear_strategy.max_speed_shift_increment(current_gear_index);
		desired_shift_reason = 4;
	end
end

if (gear_spd_radps(current_gear_index) < gear_strategy.min_speed_radps(current_gear_index)) && ( command_gear_num > gear_strategy.launch_gear_num)
    desired_gear_num = command_gear_num - gear_strategy.min_speed_shift_increment(current_gear_index);
    desired_shift_reason = 5;
end

if vehicle_spd_mps <= 1
    desired_gear_num = gear_strategy.launch_gear_num;
    desired_shift_reason = 6;
end

desired_gear_num = min(num_gear_indices-1 , max(1, desired_gear_num));

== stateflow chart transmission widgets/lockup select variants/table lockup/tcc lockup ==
  state TCC_OFF
    entry:
    tcc_lockup = false;
    timer = 0;
    during:
    timer += step_time;
  state TCC_ON
    entry:
    tcc_lockup=true;
  (default) -> TCC_OFF
  TCC_OFF -> TCC_OFF : [lock_spd < lockup_spd || ... ~lockup_allowed]
  TCC_OFF -> TCC_ON : [lockup_allowed && ... (lock_spd >= lockup_spd) && ...  (timer >= lockup_delay_secs)]
  TCC_ON -> TCC_OFF : [lock_spd <= release_spd]
